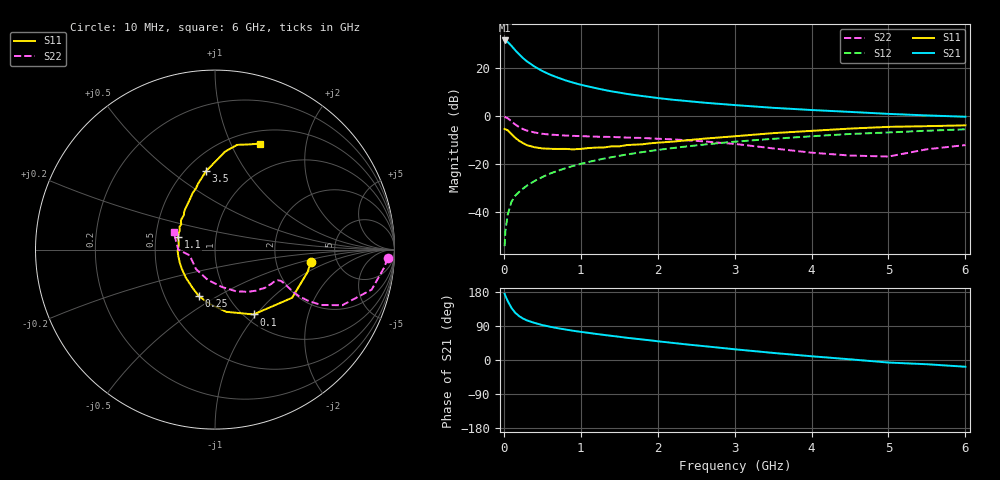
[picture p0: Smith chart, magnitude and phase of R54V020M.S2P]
! SIEMENS Small Signal Semiconductors
! BFR183
! Si NPN RF Bipolar Junction Transistor in SOT23
! VCE = 4 V  IC = 20 mA
! Common Emitter S-Parameters:  May  1996
# GHz  S  MA  R  50
!  f  S11  S21  S12  S22
! GHz  MAG  ANG  MAG  ANG  MAG  ANG  MAG  ANG
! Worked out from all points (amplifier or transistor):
!   36 points, 10 MHz to 6 GHz, reference 50 ohm
!   highest |S21| = 31.3 dB at 10 MHz (marker M1)
!   |S21| within 3 dB of that: start of sweep to 119.8 MHz
!   unconditionally stable (mu >= 1): 577.9 MHz to 2.376 GHz
!   at 250 MHz: K = 0.81, MSG = 27.1 dB, |S12| = -30.1 dB
!   at 1.4 GHz: K = 1.04, MAG = 12.4 dB, |S12| = -17.1 dB
!   at 6 GHz: K = 0.90, MSG = 2.6 dB, |S12| = -5.5 dB
!   S11 on the Smith chart (normalised r, x): 10 MHz: 3.21, -0.60; 100 MHz: 1.10, -0.97; 250 MHz: 0.74, -0.41; 1.1 GHz: 0.65, +0.09; 3.5 GHz: 0.62, +0.68; 6 GHz: 0.65, +1.29
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0.01  0.5385 -7.1  36.93 174.6  0.002 88.7  0.9627 -2.8
0.02  0.5312 -13.5  36.37 169.5  0.0041 82.4  0.9483 -6.0
0.05  0.5067 -32.0  34.34 155.7  0.009 76.9  0.9011 -14.3
0.1  0.4202 -59.3  28.45 137.3  0.0168 71.4  0.7739 -23.6
0.15  0.3524 -79.7  22.98 124.2  0.0225 68.5  0.6656 -27.6
0.2  0.3046 -95.4  18.97 115.6  0.0267 68.6  0.5895 -28.8
0.25  0.274 -109.3  15.87 109.3  0.0313 68.3  0.5344 -29.0
0.3  0.2486 -119.7  13.62 104.5  0.036 69.4  0.4995 -28.5
0.4  0.2252 -136.5  10.59 97.8  0.045 70.2  0.4555 -27.1
0.5  0.2131 -150.9  8.584 92.2  0.0543 71.3  0.4281 -26.0
0.6  0.2092 -160.6  7.235 87.8  0.064 71.7  0.4127 -25.5
0.7  0.2076 -170.7  6.274 83.9  0.0732 71.4  0.4029 -25.5
0.8  0.2084 -178.4  5.504 80.5  0.0827 70.8  0.3941 -25.8
0.9  0.2035 174.0  4.924 77.2  0.0923 70.5  0.3877 -26.1
1.1  0.2167 161.6  4.094 71.6  0.1115 69.5  0.3786 -27.9
1.3  0.2228 151.8  3.491 66.2  0.1308 67.8  0.3704 -29.8
1.6  0.2505 139.4  2.877 58.6  0.1596 65.0  0.3572 -34.1
2.2  0.2945 121.5  2.175 45.0  0.2171 58.8  0.328 -44.0
3.5  0.4418 96.3  1.481 18.7  0.3368 42.6  0.2132 -78.8
4.5  0.5492 84.1  1.218 1.8  0.4245 30.0  0.1516 -134.3
5.5  0.6164 72.0  1.029 -11.2  0.496 18.2  0.2046 179.9
6  0.6406 67.1  0.967 -17.8  0.5298 10.7  0.2499 157.2
